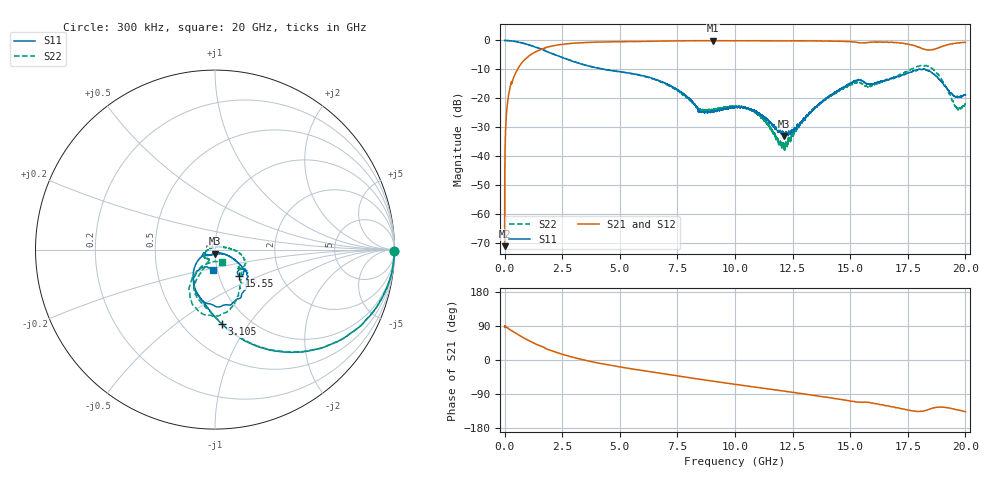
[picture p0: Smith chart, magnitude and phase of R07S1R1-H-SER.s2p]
!{R07S1R1}
!Johanson Technology Inc.
!www.johansontechnology.com
!Test Board Conditions:
!Substrate Type  RO4350B
!Substrate Thickness  10 mil
!Substrate Dk  3.66
!TL Type: GCPW
!TL Trace Width  21 mil
!TL Gap  20 mil
!Electrode orientation  Horizontal
!DUT TOPOLOGY	SERIES
!Mounting Pad LxW  16x21 mil
! Created Fri Feb  5 23:10:00 2021
# hz S ma R 50
! 2 Port Network Data from SP1.SP block
! freq  magS11  angS11  magS21  angS21  magS12  angS12  magS22  angS22
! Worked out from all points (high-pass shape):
!   20001 points, 300 kHz to 20 GHz, reference 50 ohm
!   highest |S21| = -0.07 dB at 9.059 GHz (marker M1); lowest = -71.1 dB at 300 kHz (marker M2)
!   |S21| within 3 dB of the highest: 1.598 GHz to 18.24 GHz (16.64 GHz wide, 168 % of centre); 18.63 GHz to end of sweep
!   lowest |S11| = -32.9 dB at 12.14 GHz (marker M3), VSWR 1.05, Z = 50.1 - j2.25 ohm
!   |S11| at or under -10 dB: 4.341 GHz to 17.97 GHz (13.63 GHz wide, 122 % of centre); 18.0626 GHz to 18.13509 GHz (72.49 MHz wide, 0.401 % of centre); 18.25 GHz to end of sweep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
!   |S22| runs from -38.0 to 0.0 dB; largest |S21 - S12| = 0.012
!   S11 on the Smith chart (normalised r, x): 300 kHz: open; 3.105 GHz: 0.75, -0.76; 15.55 GHz: 1.25, -0.38; 20 GHz: 0.96, -0.22
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300000  1 -0.5  0.0002802 85.9  0.0003249 75.8  0.9995 -0.5
1.013e8  0.9955 -4.5  0.06702 85.8  0.06711 85.8  0.9966 -4.4
1.363e8  0.9956 -6.1  0.09008 84.3  0.09004 84.3  0.995 -6.1
2.583e8  0.9839 -11.4  0.1688 79.3  0.1687 79.2  0.9839 -11.3
4.993e8  0.9561 -19.6  0.2866 70.2  0.2864 70.1  0.9565 -19.4
1.4833e9  0.7304 -51.3  0.6747 38.8  0.6744 38.7  0.7363 -50.8
3.1053e9  0.4179 -84.5  0.9038 5.0  0.9021 5.0  0.4198 -84.2
3.3343e9  0.3914 -87.7  0.9146 1.6  0.9142 1.6  0.3932 -87.5
6.6673e9  0.2055 -126.5  0.9738 -34.1  0.9742 -34.2  0.2005 -121.2
8.4873e9  0.05904 -157.8  0.9896 -50.9  0.9905 -51.0  0.06464 -121.5
9.0593e9  0.05866 -160.8  0.9923 -56.1  0.9905 -56.1  0.06339 -127.7
1.00003e10  0.07096 -157.7  0.9899 -64.2  0.99 -64.3  0.07206 -144.9
1.09953e10  0.05483 -146.0  0.9889 -72.5  0.9868 -72.6  0.05255 -167.7
1.21423e10  0.02253 -86.8  0.986 -82.2  0.9871 -82.3  0.01389 98.7
1.33343e10  0.06042 -24.7  0.9821 -92.5  0.9822 -92.6  0.06162 9.6
1.55493e10  0.2005 -47.4  0.9075 -111.4  0.9058 -111.2  0.1758 -38.7
1.66673e10  0.2085 -34.8  0.9235 -121.4  0.9281 -121.7  0.2133 -46.5
1.76423e10  0.2838 -56.4  0.8409 -133.6  0.8436 -133.8  0.3205 -69.9
1.83493e10  0.3027 -96.8  0.6848 -131.6  0.6851 -131.9  0.3619 -101.6
1.88953e10  0.2066 -125.5  0.7619 -124.2  0.761 -124.1  0.2355 -125.6
1.96133e10  0.1061 -113.1  0.904 -131.2  0.9046 -130.9  0.0704 -99.6
2e10  0.1156 -94.3  0.9283 -136.3  0.9235 -136.2  0.08191 -58.2
